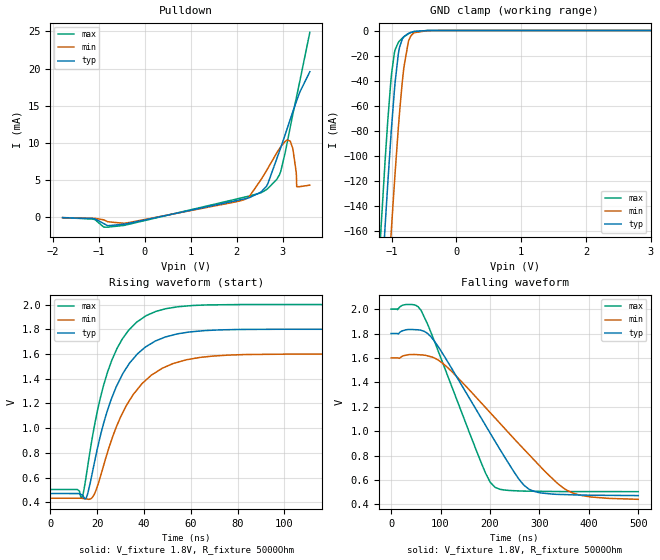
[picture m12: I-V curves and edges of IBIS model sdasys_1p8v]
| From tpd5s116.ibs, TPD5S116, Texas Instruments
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[Model]   sdasys_1p8v
Model_type   I/O_open_drain
Polarity   Non-Inverting
Enable   Active-Low
Vinl = .1312
Vinh = 1.4
Vmeas = 0.9
Vref = 1.8
Cref = 15pF
Rref = 5000
|   typ   min   max
|   (nom PVT)   (slow PVT)   (fast PVT)
C_comp   1.0804p   0.9332p   1.0809p
| Where nom  PVT is Nominal Process, 1.8V, 27C
|   Fast PVT is Strong Process,  2.0V, -40C
|   Slow PVT is Weak Process,   1.6V, 125C
[Voltage Range]   1.8   1.6   2
[Temperature Range]   27   125   -40
[Pullup Reference]   1.8   1.6   2
[Pulldown Reference]   -0   -0   -0
[Power Clamp Reference]   1.8   1.6   2
[GND Clamp Reference]   -0   -0   -0
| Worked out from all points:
|   slope of the pulldown table from 0 to 0.27 V, typ, clamps not added: 766 ohm
|   GND clamp passes 1 mA (typ) near -0.67 V on its own axis
|   falling waveform, V_fixture 1.8V, R_fixture 5000Ohm: 20-80 % time 118ns typ, 159ns min, 85.1ns max; typ from 1.8 V to 0.473 V
|   rising waveform, V_fixture 1.8V, R_fixture 5000Ohm: 20-80 % time 15.1ns typ, 17.2ns min, 13.3ns max; typ from 0.472 V to 1.8 V
[Pulldown]
|   Voltage   I(typ)   I(min)   I(max)
-1.789V   -41.79uA   -40.83uA   -41.22uA
-1.13V    -168.7uA   -123.6uA   -229.2uA
-806.4mV  -1.125mA   -590.9uA   -1.32mA
2.045V    2.317mA    2.17mA     2.53mA
2.266V    2.618mA    2.709mA    2.851mA
2.65V     4.176mA    6.254mA    3.73mA
2.936V    8.937mA    9.263mA    5.754mA
3.103V    11.98mA    10.39mA    10.09mA
3.227V    14.27mA    9.126mA    13.95mA
3.298V    15.52mA    6.081mA    15.98mA
3.308V    15.71mA    4.13mA     16.3mA
3.595V    19.58mA    4.331mA    24.88mA
[GND Clamp]
|   Voltage   I(typ)   I(min)   I(max)
-1.789V   -799mA     -881.7mA   -747.6mA
-1.184V   -228.7mA   -314.1mA   -174.8mA
-1.103V   -158.1mA   -242.5mA   -105.6mA
-1.06V    -122.3mA   -205.4mA   -72.03mA
-1.006V   -80.46mA   -160.4mA   -36.98mA
-957.6mV  -47.72mA   -121.9mA   -17.78mA
-887.4mV  -15.85mA   -71.46mA   -8.882mA
-811.8mV  -4.886mA   -29.51mA   -5.097mA
-741.6mV  -2.304mA   -8.802mA   -2.616mA
-655.2mV  -830uA     -1.781mA   -803.4uA
-450mV    -20.57uA   -66.55uA   -8.889uA
3.595V    0A         0A         0A
[Ramp]
R_load = 5000
|   typ   min   max
dV/dt_r   0.794853/1.50822e-08   0.69986/1.72536e-08   0.897091/1.32534e-08
dV/dt_f   0.796443/1.17828e-07   0.694835/1.59195e-07   0.897007/8.51306e-08
[Falling Waveform]
V_fixture = 1.8V
V_fixture_min = 1.6V
V_fixture_max = 2V
R_fixture = 5000Ohm
C_fixture = 0F
|   Time   V(typ)   V(min)   V(max)
0s        1.8V       1.6V       2V
41ns      1.833V     1.628V     2.038V
60.85ns   1.826V     1.625V     1.988V
105.6ns   1.627V     1.552V     1.548V
190.6ns   1.051V     1.196V     661.1mV
210.6ns   915.6mV    1.107V     539.8mV
258.5ns   607.5mV    896.1mV    510.7mV
288.5ns   507.5mV    767.7mV    508.3mV
365.3ns   479.1mV    497.4mV    505.5mV
500ns     472.6mV    441.9mV    505mV
[Rising Waveform]
V_fixture = 1.8V
V_fixture_min = 1.6V
V_fixture_max = 2V
R_fixture = 5000Ohm
C_fixture = 0F
|   Time   V(typ)   V(min)   V(max)
0s        471.8mV    433.8mV    504.6mV
13.54ns   461.2mV    433.1mV    438.9mV
15.47ns   442.2mV    427.6mV    629.2mV
18.84ns   721.5mV    466.8mV    1.018V
22.71ns   1.035V     694.2mV    1.343V
28.47ns   1.347V     1.022V     1.643V
39.27ns   1.634V     1.362V     1.888V
54.59ns   1.764V     1.534V     1.982V
105.6ns   1.8V       1.6V       2V
500ns     1.797V     1.6V       2V
